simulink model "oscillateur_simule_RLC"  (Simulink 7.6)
settings: Solver=ode14x  StartTime=0.0  StopTime=N  RelTol=1e-3
InitFcn:
  | clear all, clc
  | N=2;
  | R1=1e3;
  | R2=R1;
  | R=R1;
  | C=10e-3;
StopFcn:
  | close all, clc
  | load oscillateur_LC.mat
  | plot(x(1,:),x(2,:))
  | title('Signal de sortie de l''oscillateur RLC et résistance négative')
  | %axis([0 N -1.5e-8 1.5e-8])
  | xlabel('temps')
  | grid
libraries: fl_lib x16, nesl_utility x4, elec_lib x4, simulink x1

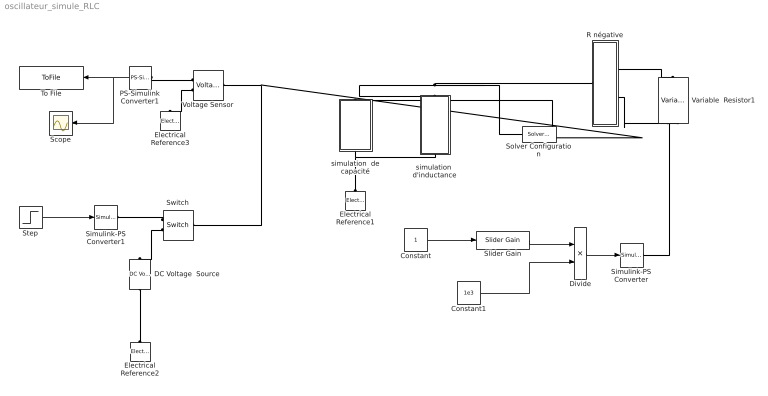
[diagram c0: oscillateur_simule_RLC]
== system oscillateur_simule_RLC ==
  Constant : Constant
  Constant1 : Constant  Value=1e3
  DC Voltage  Source : fl_lib/Electrical/Electrical Sources/DC Voltage Source  DialogController=NetworkEngine.DynNeDlgSource  SystemSampleTime=-1  v0=0.1 V  i_Log=off  v_Log=off  LocalVarNames=|i|v  LocalVarDescs=|i|v  LocalVarLogging=[0 0]
  Divide : Product  Inputs=**
  Electrical Reference1 : fl_lib/Electrical/Electrical Elements/Electrical Reference  DialogController=NetworkEngine.DynNeDlgSource  SystemSampleTime=-1  i_Log=off  LocalVarNames=|i  LocalVarDescs=|i  LocalVarLogging=[]
  Electrical Reference2 : fl_lib/Electrical/Electrical Elements/Electrical Reference  DialogController=NetworkEngine.DynNeDlgSource  SystemSampleTime=-1  i_Log=off  LocalVarNames=|i  LocalVarDescs=|i  LocalVarLogging=[]
  Electrical Reference3 : fl_lib/Electrical/Electrical Elements/Electrical Reference  DialogController=NetworkEngine.DynNeDlgSource  SystemSampleTime=-1  i_Log=off  LocalVarNames=|i  LocalVarDescs=|i  LocalVarLogging=[]
  PS-Simulink Converter1 : nesl_utility/PS-Simulink Converter  DialogController=NetworkEngine.DynNeUtilDlgSource  SystemSampleTime=-1  PhysicalDomain=network_engine_domain  LeftPortType=input  RightPortType=output  SubClassName=ps_output  Unit=1  AffineConversion=off
  R négative : Subsystem
  Scope : Scope
  Simulink-PS Converter : nesl_utility/Simulink-PS Converter  DialogController=NetworkEngine.DynNeUtilDlgSource  SystemSampleTime=-1  PhysicalDomain=network_engine_domain  LeftPortType=input  RightPortType=output  SubClassName=ps_input  Unit=1  AffineConversion=off  InputFilterTimeConstant=.001  UdotUserProvided=0
  Simulink-PS Converter1 : nesl_utility/Simulink-PS Converter  DialogController=NetworkEngine.DynNeUtilDlgSource  SystemSampleTime=-1  PhysicalDomain=network_engine_domain  LeftPortType=input  RightPortType=output  SubClassName=ps_input  Unit=1  AffineConversion=off  InputFilterTimeConstant=.001  UdotUserProvided=0
  Slider Gain : simulink/Math Operations/Slider Gain  SystemSampleTime=-1  low=0  gain=0.5  high=1.1438
  Solver Configuration : nesl_utility/Solver Configuration  DialogController=NetworkEngine.DynNeUtilDlgSource  SystemSampleTime=-1  PhysicalDomain=network_engine_domain  LeftPortType=input  RightPortType=generic  SubClassName=solver  Accelerate=off  Profile=off  ResidualTolerance=1e-9  MaxNonlinIter=12  MaxModeIter=2  DoFixedCost=off  UseLocalSampling=off  DoDC=off  LinearAlgebra=Sparse  LocalSolverSampleTime=.001  LocalSolverChoice=NE_BACKWARD_EULER_ADVANCER  UseLocalSolver=off
  Step : Step  Time=0.1  Before=10  After=0  SampleTime=0
  Switch : fl_lib/Electrical/Electrical Elements/Switch  DialogController=NetworkEngine.DynNeDlgSource  SystemSampleTime=-1  R_closed=0.01 Ohm  G_open=1e-08 1/Ohm  Threshold=0.5  i_Log=off  v_Log=off  LocalVarNames=|i|v  LocalVarDescs=|i|v  LocalVarLogging=[0 0]
  To File : ToFile  Filename=oscillateur_LC  MatrixName=x
  Variable  Resistor1 : fl_lib/Electrical/Electrical Elements/Variable Resistor  DialogController=NetworkEngine.DynNeDlgSource  SystemSampleTime=-1  Rmin=0 Ohm  i_Log=off  v_Log=off  LocalVarNames=|i|v  LocalVarDescs=|i|v  LocalVarLogging=[0 0]
  Voltage Sensor : fl_lib/Electrical/Electrical Sensors/Voltage Sensor  DialogController=NetworkEngine.DynNeDlgSource  SystemSampleTime=-1  i1_Log=off  v1_Log=off  LocalVarNames=|i1|v1  LocalVarDescs=|i1|v1  LocalVarLogging=[0 0]
  simulation  d'inductance : Subsystem
  simulation  de capacité : Subsystem
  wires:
  PS-Simulink Converter1/1 -> To File/1, Scope/1
  Step/1 -> Simulink-PS Converter1/1
  Constant/1 -> Slider Gain/1
  Slider Gain/1 -> Divide/1
  Constant1/1 -> Divide/2
  Divide/1 -> Simulink-PS Converter/1
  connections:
  Voltage Sensor/RConn2 -- Electrical Reference3/LConn1
  PS-Simulink Converter1/LConn1 -- Voltage Sensor/RConn1
  simulation  d'inductance/RConn1 -- simulation  de capacité/LConn1 -- Electrical Reference1/LConn1
  Switch/LConn1 -- simulation  d'inductance/LConn1 -- Solver Configuration/RConn1 -- R négative/LConn1 -- simulation  de capacité/RConn1 -- Voltage Sensor/LConn1
  Switch/RConn1 -- Simulink-PS Converter1/RConn1
  Electrical Reference2/LConn1 -- DC Voltage  Source/RConn1
  Switch/RConn2 -- DC Voltage  Source/LConn1
  R négative/RConn1 -- Variable  Resistor1/RConn1
  R négative/RConn2 -- Variable  Resistor1/LConn2
  Simulink-PS Converter/RConn1 -- Variable  Resistor1/LConn1

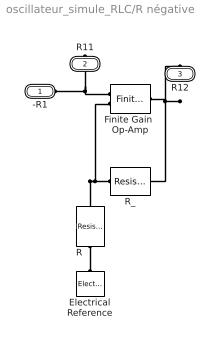
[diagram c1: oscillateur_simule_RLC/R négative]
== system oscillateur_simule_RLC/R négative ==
  Electrical Reference : fl_lib/Electrical/Electrical Elements/Electrical Reference  DialogController=NetworkEngine.DynNeDlgSource  SystemSampleTime=-1  i_Log=off  LocalVarNames=|i  LocalVarDescs=|i  LocalVarLogging=0
  Finite Gain  Op-Amp : elec_lib/Integrated Circuits/Finite Gain Op-Amp  DialogController=NetworkEngine.DynNeDlgSource  SystemSampleTime=-1  A=1000  Rin=1e+6 Ohm  Rout=100 Ohm  Vmin=-15 V  Vmax=15 V  LocalVarLogging=[]
  R : fl_lib/Electrical/Electrical Elements/Resistor  DialogController=NetworkEngine.DynNeDlgSource  SystemSampleTime=-1  R=1 kOhm  i_Log=off  v_Log=off  LocalVarNames=|i|v  LocalVarDescs=|i|v  LocalVarLogging=[0 0]
  R_ : fl_lib/Electrical/Electrical Elements/Resistor  DialogController=NetworkEngine.DynNeDlgSource  SystemSampleTime=-1  R=1 kOhm  i_Log=off  v_Log=off  LocalVarNames=|i|v  LocalVarDescs=|i|v  LocalVarLogging=[0 0]
  -R1 : PMIOPort  Port=1  Side=Left
  R11 : PMIOPort  Port=2  Side=Right
  R12 : PMIOPort  Port=3  Side=Right
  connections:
  R/RConn1 -- Electrical Reference/LConn1
  R11/RConn1 -- -R1/RConn1 -- Finite Gain  Op-Amp/LConn1
  R_/LConn1 -- Finite Gain  Op-Amp/LConn2 -- R/LConn1
  Finite Gain  Op-Amp/RConn1 -- R12/RConn1 -- R_/RConn1

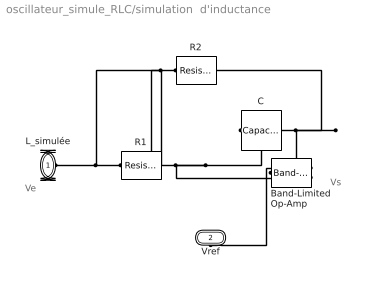
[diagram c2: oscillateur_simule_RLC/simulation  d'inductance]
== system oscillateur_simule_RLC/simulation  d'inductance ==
  note: Vs
  note: Ve
  Band-Limited Op-Amp : elec_lib/Integrated Circuits/Band-Limited Op-Amp  DialogController=NetworkEngine.DynNeDlgSource  SystemSampleTime=-1  A=1000  Rin=1e+6 Ohm  Rout=100 Ohm  Vmin=-15 V  Vmax=15 V  Vdotmax=1000 V/s  f=1e+5 Hz  V0=0 V  LocalVarLogging=[]
  C : fl_lib/Electrical/Electrical Elements/Capacitor  DialogController=NetworkEngine.DynNeDlgSource  SystemSampleTime=-1  c=C F  v0=0 V  r=1e-22 Ohm  g=0 1/Ohm  i_Log=off  v_Log=off  vc_Log=off  LocalVarNames=|i|v|vc  LocalVarDescs=|i|v|Internal variable for voltage across capacitor term  LocalVarLogging=[0 0 0]
  R1 : fl_lib/Electrical/Electrical Elements/Resistor  DialogController=NetworkEngine.DynNeDlgSource  SystemSampleTime=-1  R=R1 Ohm  i_Log=off  v_Log=off  LocalVarNames=|i|v  LocalVarDescs=|i|v  LocalVarLogging=[0 0]
  R2 : fl_lib/Electrical/Electrical Elements/Resistor  DialogController=NetworkEngine.DynNeDlgSource  SystemSampleTime=-1  R=R2 Ohm  i_Log=off  v_Log=off  LocalVarNames=|i|v  LocalVarDescs=|i|v  LocalVarLogging=[0 0]
  L_simulée : PMIOPort  Port=1  Side=Left
  Vref : PMIOPort  Port=2  Side=Right
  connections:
  R1/LConn1 -- C/RConn1 -- Band-Limited Op-Amp/LConn2
  C/LConn1 -- R2/RConn1 -- Band-Limited Op-Amp/RConn1
  R2/LConn1 -- L_simulée/RConn1 -- R1/RConn1
  Band-Limited Op-Amp/LConn1 -- Vref/RConn1

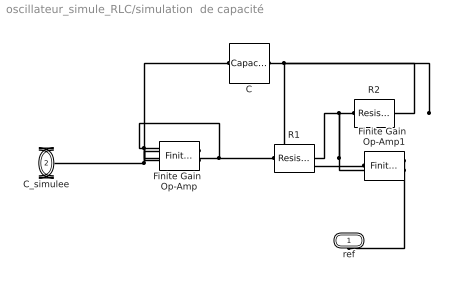
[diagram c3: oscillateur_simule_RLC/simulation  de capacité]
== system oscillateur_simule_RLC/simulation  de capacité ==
  C : fl_lib/Electrical/Electrical Elements/Capacitor  DialogController=NetworkEngine.DynNeDlgSource  SystemSampleTime=-1  c=C F  v0=0 V  r=1e-22 Ohm  g=0 1/Ohm  i_Log=off  v_Log=off  vc_Log=off  LocalVarNames=|i|v|vc  LocalVarDescs=|i|v|Internal variable for voltage across capacitor term  LocalVarLogging=[0 0 0]
  Finite Gain  Op-Amp : elec_lib/Integrated Circuits/Finite Gain Op-Amp  DialogController=NetworkEngine.DynNeDlgSource  SystemSampleTime=-1  A=1000  Rin=1e+6 Ohm  Rout=100 Ohm  Vmin=-15 V  Vmax=15 V  LocalVarLogging=[]
  Finite Gain  Op-Amp1 : elec_lib/Integrated Circuits/Finite Gain Op-Amp  DialogController=NetworkEngine.DynNeDlgSource  SystemSampleTime=-1  A=1000  Rin=1e+6 Ohm  Rout=100 Ohm  Vmin=-15 V  Vmax=15 V  LocalVarLogging=[]
  R1 : fl_lib/Electrical/Electrical Elements/Resistor  DialogController=NetworkEngine.DynNeDlgSource  SystemSampleTime=-1  R=R1 Ohm  i_Log=off  v_Log=off  LocalVarNames=|i|v  LocalVarDescs=|i|v  LocalVarLogging=[0 0]
  R2 : fl_lib/Electrical/Electrical Elements/Resistor  DialogController=NetworkEngine.DynNeDlgSource  SystemSampleTime=-1  R=R2 Ohm  i_Log=off  v_Log=off  LocalVarNames=|i|v  LocalVarDescs=|i|v  LocalVarLogging=[0 0]
  ref : PMIOPort  Port=1  Side=Right
  C_simulee : PMIOPort  Port=2  Side=Left
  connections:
  Finite Gain  Op-Amp1/LConn1 -- ref/RConn1
  C/LConn1 -- Finite Gain  Op-Amp1/RConn1 -- R2/RConn1
  C/RConn1 -- Finite Gain  Op-Amp/LConn1 -- C_simulee/RConn1
  R2/LConn1 -- Finite Gain  Op-Amp1/LConn2 -- R1/RConn1
  Finite Gain  Op-Amp/LConn2 -- R1/LConn1 -- Finite Gain  Op-Amp/RConn1
